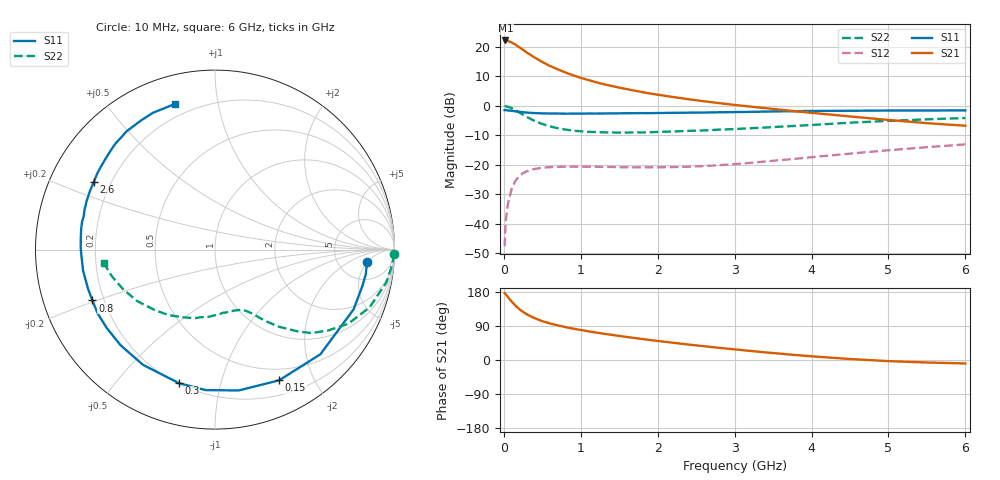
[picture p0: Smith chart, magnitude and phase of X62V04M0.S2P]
! SIEMENS Small Signal Semiconductors
! BFP193W
! Si NPN RF Bipolar Junction Transistor in SOT343
! VCE = 2 V  IC = 4 mA
! Common Emitter S-Parameters:  April 1994
# GHz  S  MA  R  50
!  f  S11  S21  S12  S22
! GHz  MAG  ANG  MAG  ANG  MAG  ANG  MAG  ANG
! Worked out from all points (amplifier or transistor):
!   40 points, 10 MHz to 6 GHz, reference 50 ohm
!   highest |S21| = 22.2 dB at 20 MHz (marker M1)
!   |S21| within 3 dB of that: start of sweep to 240.7 MHz
!   unconditionally stable (mu >= 1): 1.783 GHz to 4.624 GHz
!   at 200 MHz: K = 0.12, MSG = 21.9 dB, |S12| = -23.8 dB
!   at 1.5 GHz: K = 0.87, MSG = 13.5 dB, |S12| = -20.8 dB
!   at 6 GHz: K = 0.95, MSG = 3.2 dB, |S12| = -13.0 dB
!   S11 on the Smith chart (normalised r, x): 10 MHz: 10, -5; 150 MHz: 0.36, -1.54; 300 MHz: 0.20, -0.75; 800 MHz: 0.16, -0.19; 2.6 GHz: 0.14, +0.25; 6 GHz: 0.14, +0.76
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0.01  0.85 -4.6  12.85 176.6  0.0042 87.6  0.9979 -1.4
0.02  0.8512 -9.4  12.89 174.7  0.0087 84.1  0.9908 -4.6
0.03  0.8458 -13.9  12.85 172.1  0.0128 82.5  0.9847 -6.6
0.05  0.841 -23.3  12.66 166.8  0.0209 78.4  0.9717 -10.9
0.1  0.8276 -44.8  11.94 154.6  0.0387 67.2  0.9194 -20.5
0.15  0.8112 -63.9  10.99 143.5  0.0536 57.5  0.8496 -29.1
0.2  0.7958 -80.4  9.909 134.4  0.0647 49.9  0.7755 -35.5
0.25  0.7846 -93.8  8.952 126.9  0.0727 43.5  0.7104 -40.9
0.3  0.7708 -105.1  8.029 120.4  0.0783 38.8  0.6479 -44.7
0.4  0.757 -122.1  6.617 110.3  0.0856 31.3  0.5574 -50.4
0.5  0.7488 -134.7  5.558 102.6  0.0896 26.5  0.4948 -54.2
0.6  0.7447 -144.1  4.766 96.5  0.0917 23.0  0.4507 -57.1
0.8  0.7395 -157.5  3.69 86.9  0.0934 19.2  0.3981 -61.3
1.1  0.7444 -171.1  2.749 75.7  0.0935 16.6  0.3643 -67.1
1.3  0.7456 -178.2  2.338 69.3  0.0927 16.3  0.3571 -71.5
1.6  0.7521 173.3  1.927 60.6  0.0915 17.7  0.354 -77.8
2.2  0.7648 159.2  1.418 45.5  0.0919 23.7  0.3683 -91.8
2.6  0.773 151.0  1.203 36.4  0.0957 29.0  0.3842 -101.5
3.2  0.7938 139.8  0.977 24.1  0.1084 36.0  0.418 -115.6
4.5  0.829 120.0  0.664 2.6  0.1556 41.1  0.5199 -146.5
5.5  0.8366 109.9  0.511 -6.6  0.2 38.0  0.5934 -165.5
6  0.842 105.2  0.462 -9.1  0.2233 35.8  0.6243 -173.1
